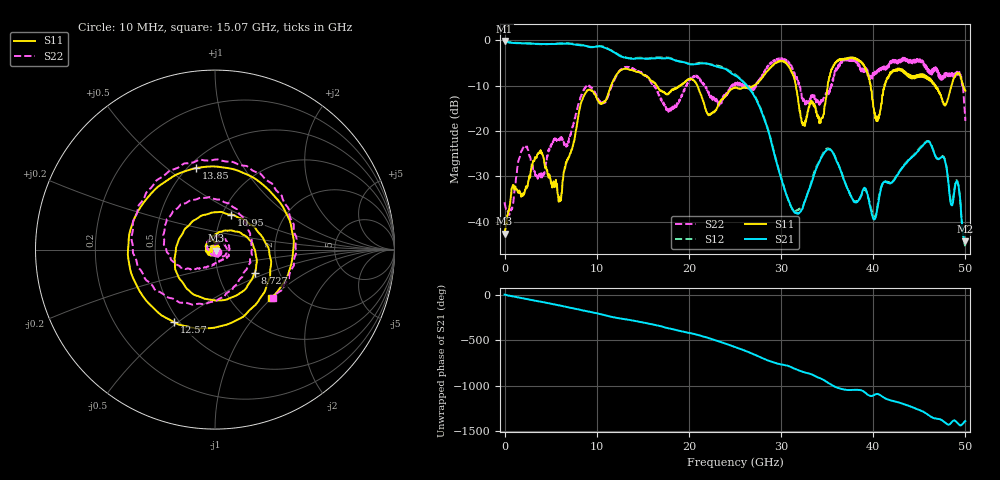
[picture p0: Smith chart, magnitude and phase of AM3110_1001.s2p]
# Hz S DB R 50.0
!freq dBS11 angS11 dBS21 angS21 dBS12 angS12 dBS22 angS22
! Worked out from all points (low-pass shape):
!   1601 points, 10 MHz to 50 GHz, reference 50 ohm
!   highest |S21| = -0.15 dB at 10 MHz (marker M1); lowest = -44.3 dB at 49.94 GHz (marker M2)
!   |S21| within 3 dB of the highest: start of sweep to 12.27 GHz
!   lowest |S11| = -42.6 dB at 10 MHz (marker M3), VSWR 1.01, Z = 50.5 - j0.549 ohm
!   |S11| at or under -10 dB: start of sweep to 11.55 GHz; 20.9 GHz to 27.06 GHz (6.157 GHz wide, 25.7 % of centre); 31.61 GHz to 35.06 GHz (3.455 GHz wide, 10.4 % of centre)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
!   |S22| runs from -38.5 to -3.9 dB; largest |S21 - S12| = 0.02
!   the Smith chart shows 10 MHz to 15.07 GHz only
!   S11 on the Smith chart (normalised r, x): 10 MHz: 1.01, -0.01; 8.727 GHz: 1.50, -0.42; 10.95 GHz: 1.10, +0.45; 12.57 GHz: 0.47, -0.49; 13.85 GHz: 0.55, +0.64; 15.07 GHz: 1.53, -0.99
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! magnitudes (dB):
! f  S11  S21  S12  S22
! 10 MHz  -42.6  -0.2  -0.1  -35.7
! 2.072 GHz  -34.0  -0.7  -0.7  -23.5
! 3.79 GHz  -24.6  -0.8  -0.9  -29.4
! 6.009 GHz  -35.5  -0.7  -0.7  -21.9
! 8.352 GHz  -13.5  -1.1  -1.0  -12.0
! 8.727 GHz  -11.8  -1.2  -1.1  -10.5
! 10.95 GHz  -13.4  -1.7  -1.6  -13.7
! 12.57 GHz  -6.7  -3.6  -3.4  -6.5
! 13.85 GHz  -6.6  -4.1  -4.0  -6.2
! 15.07 GHz  -7.7  -4.0  -3.9  -7.5
! 16.69 GHz  -10.6  -3.9  -3.8  -11.9
! 25 GHz  -10.5  -7.8  -7.5  -9.7
! 31.25 GHz  -7.4  -37.3  -37.3  -6.2
! 33.35 GHz  -13.5  -31.2  -30.8  -12.4
! 35.28 GHz  -8.0  -24.1  -24.0  -11.5
! 37.88 GHz  -3.8  -35.6  -35.4  -4.2
! 40.47 GHz  -17.8  -37.0  -36.3  -7.0
! 41.69 GHz  -7.9  -31.5  -31.3  -6.0
! 46.06 GHz  -8.8  -22.4  -22.3  -6.8
! 49.16 GHz  -7.2  -31.4  -31.2  -7.6
! 49.94 GHz  -11.0  -44.3  -45.1  -15.7
! 50 GHz  -11.1  -43.9  -45.4  -17.8
